PROGRAM p00_true_false
VAR
	M0: BOOL;
	M1: BOOL;
	S0: BOOL;
	L0: BOOL;
	S1: BOOL;
	L1: BOOL;
	L2: BOOL;
END_VAR

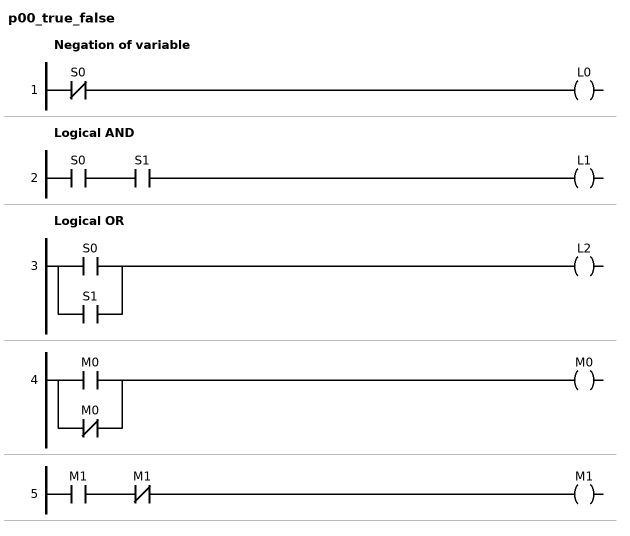
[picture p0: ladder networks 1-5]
// NETWORK 1: Negation of variable
L0 := NOT S0;

// NETWORK 2: Logical AND
L1 := S0 AND S1;

// NETWORK 3: Logical OR
L2 := S0 OR S1;

// NETWORK 4
M0 := M0 OR NOT M0;

// NETWORK 5
M1 := M1 AND NOT M1;

END_PROGRAM
